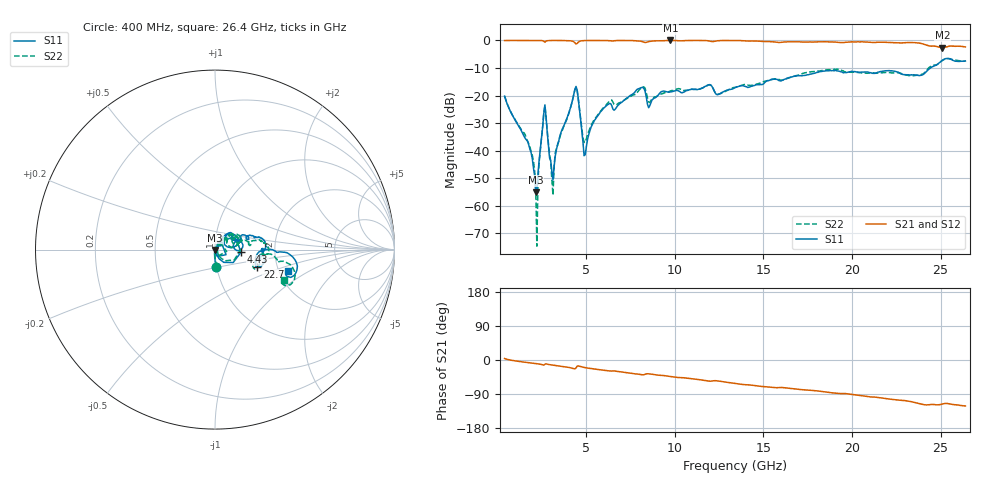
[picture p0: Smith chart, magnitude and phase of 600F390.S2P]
!  American Technical Ceramics  Date:  11/23/05
!  One Norden Lane
!  Huntington Station,  NY.  11746-2102
!  Tel:  (631) 622-4700  Fax:  (631) 622-4748
!  Part Number  600F390  Mounting Orientation: Horizontal
!  Description: Ultra Low ESR Microwave capacitors
!  Application: Coupling, Bypass, Tuning, DC Block
!  Filters, Matching
# GHZ S DB R 50
! Freq  |S11|  S11 Ph  |S21|  S21 Ph  |S12|  S12 Ph  |S22|  S22 Ph
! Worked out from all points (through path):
!   401 points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, 400 MHz to 26.4 GHz, reference 50 ohm
!   highest |S21| = 0.00 dB at 9.76 GHz (marker M1); lowest = -2.6 dB at 25.1 GHz (marker M2)
!   group delay of S21, straight-line fit = 13.1 ps
!   lowest |S11| = -55.2 dB at 2.155 GHz (marker M3), VSWR 1.00, Z = 50.1 - j0.145 ohm
!   |S11| at or under -10 dB: start of sweep to 24.43 GHz
!   |S22| runs from -74.7 to -6.5 dB; largest |S21 - S12| = 0.0078
!   S11 on the Smith chart (normalised r, x): 400 MHz: 0.99, -0.20; 4.43 GHz: 1.34, -0.04; 22.7 GHz: 1.58, -0.32; 26.4 GHz: 2.25, -0.65
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0.4  -20.22 -86.2  -0.03 3.9  -0.03 3.8  -20.22 -85.3
1.83  -39.58 -100.1  -0.01 -7.5  -0.01 -7.5  -38.75 -95.1
2.155  -55.22 -56.4  -0.01 -9.4  -0.01 -9.4  -52.76 -107.6
2.35  -43.42 52.7  -0.01 -10.7  -0.01 -10.7  -44.34 75.4
2.61  -26.45 29.3  -0.28 -13.5  -0.29 -13.4  -26.55 42.2
2.74  -27.96 -70.7  -0.23 -10.1  -0.23 -10.1  -27.97 -52.7
3  -43.58 -64.4  -0.02 -12.7  -0.03 -12.7  -44.01 -65.9
3.13  -50.67 -0.1  0.00 -13.6  -0.01 -13.6  -56.19 46.5
3.455  -36.55 58.1  0.00 -15.6  0.00 -15.6  -36.65 69.6
4.43  -16.71 -5.6  -1.28 -20.7  -1.27 -20.7  -16.94 0.5
4.755  -32.70 -67.8  -0.11 -18.3  -0.12 -18.4  -31.90 -51.4
4.95  -41.49 13.1  -0.02 -20.2  -0.03 -20.3  -37.07 10.3
6.185  -23.48 52.8  -0.03 -28.2  -0.03 -28.2  -22.97 50.4
8.07  -17.22 35.7  -0.26 -38.5  -0.25 -38.5  -17.50 38.7
9.11  -19.47 51.6  -0.16 -40.2  -0.16 -40.2  -19.74 43.4
9.76  -18.71 37.0  0.00 -43.6  -0.01 -43.5  -18.35 43.9
13.4  -17.15 22.4  -0.01 -61.7  -0.01 -61.8  -17.02 28.3
17.755  -12.11 16.2  -0.58 -80.4  -0.58 -80.5  -11.35 8.4
22.11  -10.95 -14.9  -0.75 -103.0  -0.75 -103.0  -11.68 -18.4
22.695  -11.88 -22.1  -0.91 -105.9  -0.92 -105.9  -11.81 -24.5
25.1  -7.23 -5.4  -2.60 -116.2  -2.61 -116.0  -7.25 -11.5
26.4  -7.44 -16.1  -2.36 -121.1  -2.36 -121.0  -7.50 -23.8
